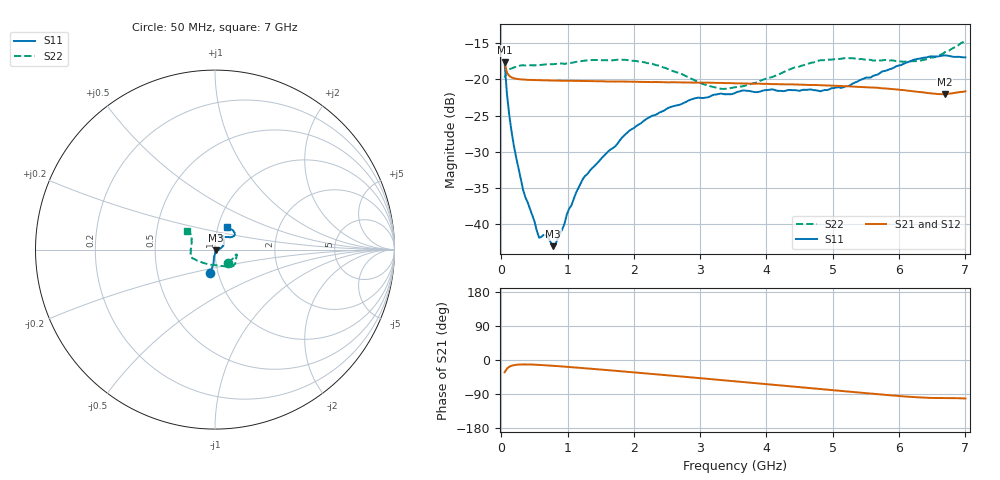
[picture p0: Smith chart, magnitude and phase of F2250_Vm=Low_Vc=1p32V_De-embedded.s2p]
! Integrated Device Technology
! Corporate Headquarters
! 6024 Silver Creek Valley Road
! San Jose, CA 95138  USA
! Phone:  1-408-284-8200
! Toll Free:  1-800-223-1366
! Webpage:  http://www.idt.com/
! Timing and RF Division
! 515 Groton Road, Suite 102
! Westford, MA 01886-6024
! Device:  F2250
! Description: Voltage Variable RF Attenuator
! Frequency:  50.0 -  6000.00 MHz
! Package:  3x3 mm Thin QFN Plastic Package: 16 pin
! Ports:  2 RF, 3 DC
!  Pin  1  = GND
!  Pin  2  = NC
!  Pin  3  = RF1  = Port 1
!  Pin  4  = NC
!  Pin  5  = GND
!  Pin  6  = GND
!  Pin  7  = GND
!  Pin  8  = GND
!  Pin  9  = NC
!  Pin 10  = RF2  = Port 2
!  Pin 11  = NC
!  Pin 12  = GND
!  Pin 13  = GND
!  Pin 14  = VCNTRL
!  Pin 15  = VDD
!  Pin 16  = VMODE
! Vcntrl:  1.320 Volts
! Vmode:  +0.000 Volts
! Vdd:  +3.30  Volts
! Current:  1.193 mA
! Data:  The device was measured on a the F2250 evaluation board which has
!  individual transmission lines to the RF pins.  Data was collected
!  using a calibrated network analyzer.  The evaluation board was
!  de-embedded using a TRL calibration technique.
!  The reference plane is the edge of the package pin.
! Misc:  SN 10
!  Action Tracker AT0258
! Date Measured:  2014-11-26
! Date:  2015-10-15  MJV
! Note:
!  Integrated Device Technology supplies this data as a sample of measured
!  data at the package pin for this product.  Your particular data for this
!  product may vary.
!  Data was taken at 25 degrees C.
!  Integrated Device Technology reserves the right to change this data at anytime.
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# GHz S dB R 50
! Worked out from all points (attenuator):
!   201 points, 50 MHz to 7 GHz, reference 50 ohm
!   highest |S21| = -17.62 dB at 50 MHz (marker M1); lowest = -22.1 dB at 6.687 GHz (marker M2)
!   lowest |S11| = -43.1 dB at 779.8 MHz (marker M3), VSWR 1.01, Z = 50.6 - j0.367 ohm
!   |S11| at or under -10 dB: start of sweep to end of sweep
!   |S22| runs from -21.3 to -14.6 dB; largest |S21 - S12| = 0.00033
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0.05  -17.64 -101.4  -17.62 -32.4  -17.62 -32.4  -19.77 -45.5
0.08475  -21.96 -96.3  -19.03 -22.9  -19.03 -22.9  -18.77 -22.7
0.15425  -27.18 -97.3  -19.71 -15.3  -19.72 -15.3  -18.48 -14.0
0.22375  -30.80 -93.4  -19.91 -12.7  -19.91 -12.7  -18.26 -13.0
0.328  -35.26 -87.5  -20.01 -11.6  -20.04 -11.6  -18.04 -13.0
0.57125  -41.94 -62.8  -20.10 -12.9  -20.12 -12.9  -18.01 -17.4
0.6755  -41.61 -51.0  -20.11 -14.0  -20.12 -14.0  -17.91 -19.8
0.77975  -43.11 -31.2  -20.16 -15.3  -20.15 -15.3  -17.88 -22.5
0.91875  -40.79 -14.5  -20.18 -17.0  -20.17 -17.0  -17.77 -26.3
1.023  -37.92 -15.9  -20.19 -18.4  -20.19 -18.4  -17.72 -27.8
1.2315  -33.77 -0.4  -20.21 -21.3  -20.21 -21.3  -17.40 -32.4
1.9265  -27.14 21.7  -20.29 -31.6  -20.30 -31.5  -17.35 -42.6
2.37825  -24.63 32.4  -20.37 -38.3  -20.36 -38.4  -18.09 -50.2
2.86475  -22.76 46.7  -20.43 -45.9  -20.43 -45.9  -19.89 -65.2
3.108  -22.48 53.8  -20.45 -49.7  -20.44 -49.7  -20.83 -78.0
3.525  -21.86 65.1  -20.53 -56.2  -20.53 -56.2  -21.08 -106.8
4.7065  -21.48 68.7  -20.76 -74.9  -20.76 -74.9  -17.64 -157.5
5.22775  -20.92 52.0  -20.94 -83.3  -20.94 -83.2  -17.05 -166.7
5.85325  -18.60 36.7  -21.30 -92.9  -21.29 -93.0  -17.37 -179.4
6.305  -17.12 37.9  -21.74 -98.8  -21.74 -98.8  -17.40 164.7
6.68725  -16.66 47.0  -22.05 -100.2  -22.04 -100.3  -16.24 149.1
7  -16.94 62.7  -21.64 -101.5  -21.63 -101.6  -14.60 145.5
